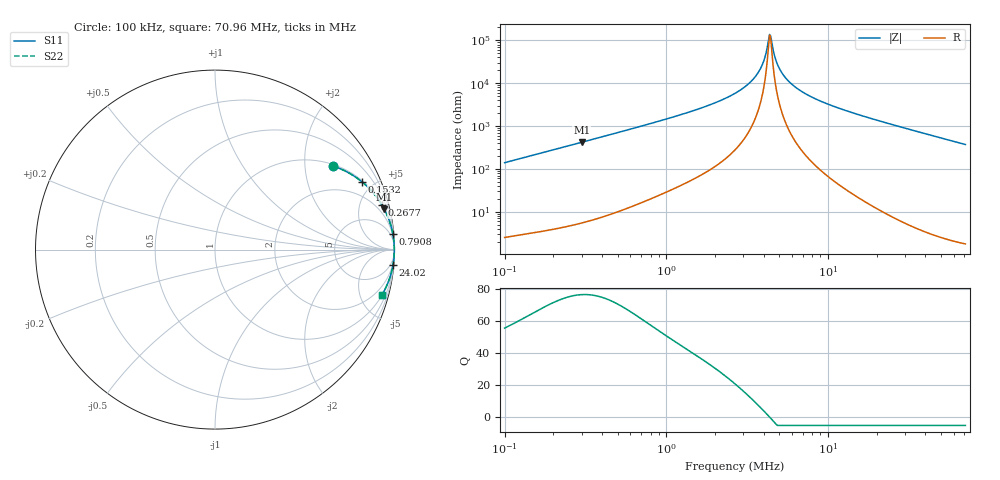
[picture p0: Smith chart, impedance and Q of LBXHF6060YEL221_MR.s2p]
! LBXHF6060YEL221_MR  S-PARAMETER MODEL  ( General Type )
! Model Generated by TAIYO YUDEN Corporation (http://www.ty-top.com)
! Version 1.0
! TAIYO YUDEN Control No. 200120NI43SB-FBB
! Copyright(c) 2020 TAIYO YUDEN CO.,LTD. All Rights Reserved.
! Product Description (link to TY-COMPAS)
! https://ds.yuden.co.jp/TYCOMPAS/or/detail?pn=LBXHF6060YEL221MMR&u=M
! Products Name : Inductors
! Characteristics :
!  Inductance : 220 uH , SRF(min) : 3.0 MHz , DC Resistance(max) : 1.32 Ohm
!  Rated Current : Saturation :700 mA , Temp Rise : 350 mA
!  Case Size : 6.0 x 6.0 / 0.236 x 0.236 [mm/inch] , Thickness : 4.5 / 0.177 [mm/inch]
!  (Conditions: Temperature = 25 degC , DC Bias Current/Voltage = 0A / 0V)
! External Node Assignments :
!  1  o---GGG---o  2
! GND o---------o GND
! Frequency Range : 0.1MHz  -  70.9631MHz  [ 402 STEP ]
# MHz S RI R 50
! Freq[MHz].  S11 Real  S11 Imag  S21 Real  S21 Imag  S12 Real  S12 Imag  S22 Real  S22 Imag
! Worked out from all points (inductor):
!   401 points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, 100 kHz to 70.96 MHz, reference 50 ohm
!   read as one part in series: L = 222 uH near 103.3 kHz
!   highest Q = 76.4 at 300.3 kHz (marker M1), where L = 223 uH
!   self-resonance near 4.359 MHz
!   S11 on the Smith chart (normalised r, x): 100 kHz: 1.05, +2.80; 153.2 kHz: 1.07, +4.28; 267.7 kHz: 1.10, +7.48; 790.8 kHz: 1, +23; 24.02 MHz: 1, -23; 70.96 MHz: 1.04, -7.44
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0.1  0.66 0.4648  0.34 -0.4648  0.34 -0.4648  0.66 0.4648
0.153221  0.8174 0.3788  0.1826 -0.3788  0.1826 -0.3788  0.8174 0.3788
0.267704  0.9305 0.2478  0.0695 -0.2478  0.0695 -0.2478  0.9305 0.2478
0.300295  0.9437 0.224  0.0563 -0.224  0.0563 -0.224  0.9437 0.224
0.790816  0.9908 0.0873  0.00922 -0.0873  0.00922 -0.0873  0.9908 0.0873
0.90177  0.9928 0.076  0.00724 -0.076  0.00724 -0.076  0.9928 0.076
1.796612  0.9979 0.0335  0.00211 -0.0335  0.00211 -0.0335  0.9979 0.0335
2.70797  0.9989 0.0166  0.00109 -0.0166  0.00109 -0.0166  0.9989 0.0166
3.243749  0.9991 0.0101  0.000869 -0.0101  0.000869 -0.0101  0.9991 0.0101
3.69886  0.9992 0.00565  0.000768 -0.00565  0.000768 -0.00565  0.9992 0.00565
4.015187  0.9993 0.00291  0.000729 -0.00291  0.000729 -0.00291  0.9993 0.00291
4.287619  0.9993 0.000726  0.000709 -0.000726  0.000709 -0.000726  0.9993 0.000726
4.358567  0.9993 0.000181  0.000706 -0.000181  0.000706 -0.000181  0.9993 0.000181
4.504005  0.9993 -0.00091  0.000702 0.00091  0.000702 0.00091  0.9993 -0.00091
4.731313  0.9993 -0.00255  0.0007 0.00255  0.0007 0.00255  0.9993 -0.00255
4.889189  0.9993 -0.00364  0.000702 0.00364  0.000702 0.00364  0.9993 -0.00364
5.395135  0.9993 -0.00696  0.000725 0.00696  0.000725 0.00696  0.9993 -0.00696
6.357379  0.9992 -0.0127  0.000821 0.0127  0.000821 0.0127  0.9992 -0.0127
7.999526  0.9989 -0.0212  0.00109 0.0212  0.00109 0.0212  0.9989 -0.0212
12.25692  0.9977 -0.0405  0.00227 0.0405  0.00227 0.0405  0.9977 -0.0405
24.02217  0.9916 -0.0875  0.00836 0.0875  0.00836 0.0875  0.9916 -0.0875
70.9631  0.9315 -0.2502  0.0685 0.2502  0.0685 0.2502  0.9315 -0.2502
